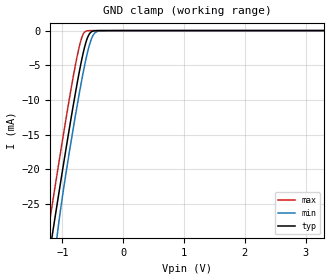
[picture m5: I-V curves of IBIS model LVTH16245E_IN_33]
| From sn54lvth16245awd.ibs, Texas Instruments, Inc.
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[Model]   LVTH16245E_IN_33
Model_type  Input
Vinl=1.05
Vinh=2.34
| variable   typ   min   max
C_comp   2.19pF   1.42pF   2.72pF
[Temperature Range]   40   100   -40
| Ambient temperature   25   85   -40
[Voltage range]   3.3   3   3.6
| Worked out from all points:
|   GND clamp passes 1 mA (typ) near -0.59 V on its own axis
[GND Clamp]
| LVTH16245E_IN_33
|   Voltage   I(typ)   I(min)   I(max)
-3.3V     -345.7mA   -367.1mA   -319mA
-1.235V   -33.48mA   -41.7mA    -28.85mA
-1.15V    -28.52mA   -34.27mA   -24.1mA
-1.095V   -25.44mA   -30.11mA   -21.05mA
-1.065V   -23.78mA   -28.03mA   -19.4mA
-935mV    -16.71mA   -20.19mA   -12.38mA
-750mV    -7.232mA   -10.42mA   -3.377mA
-680mV    -4.089mA   -7.032mA   -969uA
-615mV    -1.738mA   -4.194mA   -91.47uA
-505mV    -96.03uA   -845.6uA   -485.1nA
-385mV    -1.372uA   -34.89uA   -1.471nA
3.3V      11.84pA    1.453nA    10.54pA
